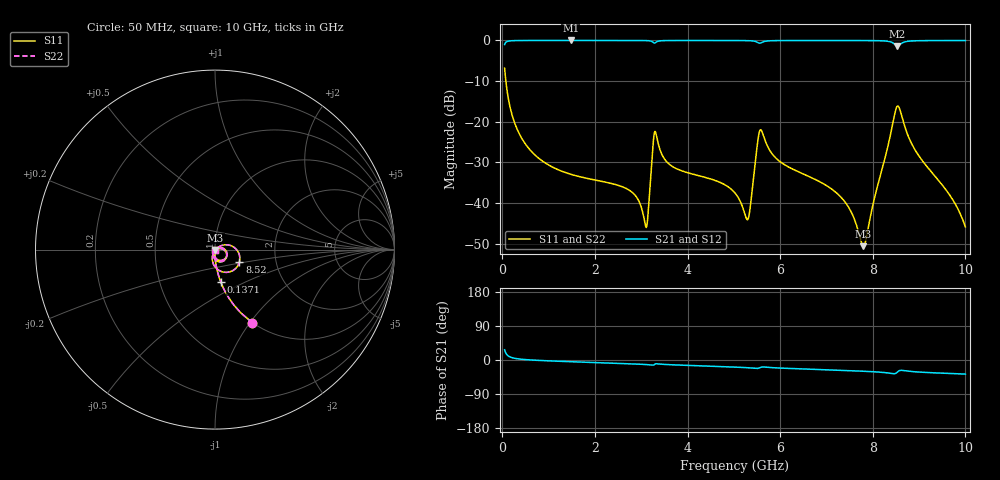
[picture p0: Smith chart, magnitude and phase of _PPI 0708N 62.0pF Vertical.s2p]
! S-Parameter data specifications (vertical orientation):
! Substrate: 40-mil Rogers 3003C, Substrate thickness, H=1.016mm, Dielectric constant, Er=3, Conductor thickness, T_mtl=0.043mm, Loss Tangent, Tand=0.003
! PCB Mounting Pad Footprint: Pad width, PadW=2.54mm , Pad length, PadL=0.51mm , Pad gap, PadG (edge-to-edge)=0.71mm , Reference planes=1.73mm apart
! Created Tue Jan 16 08:53:59 2018
# GHz S MA R 50
! 2 Port Network Data from SP1.SP block
! freq  magS11  angS11  magS21  angS21  magS12  angS12  magS22  angS22
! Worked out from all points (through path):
!   801 points, 50 MHz to 10 GHz, reference 50 ohm
!   highest |S21| = -0.01 dB at 1.48 GHz (marker M1); lowest = -1.5 dB at 8.532 GHz (marker M2)
!   group delay of S21, straight-line fit = 11.1 ps
!   lowest |S11| = -50.6 dB at 7.799 GHz (marker M3), VSWR 1.01, Z = 50.2 - j0.181 ohm
!   |S11| at or under -10 dB: 76.96 MHz to end of sweep
!   |S22| runs from -50.6 to -6.8 dB; largest |S21 - S12| = 0
!   S11 on the Smith chart (normalised r, x): 50 MHz: 1.00, -1.02; 137.1 MHz: 1.00, -0.37; 8.52 GHz: 1.30, -0.19; 10 GHz: 1.00, -0.01
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0.05  0.4558 -63.1  0.8899 26.9  0.8899 26.9  0.4558 -63.1
0.1370625  0.1841 -79.9  0.9827 10.1  0.9827 10.1  0.1841 -79.9
0.572375  0.04687 -89.2  0.9986 0.4  0.9986 0.4  0.04687 -89.2
1.480312  0.02255 -93.4  0.9992 -4.5  0.9992 -4.5  0.02255 -93.4
1.716625  0.02077 -94.2  0.9992 -5.5  0.9992 -5.5  0.02077 -94.2
2.761375  0.01412 -96.1  0.9988 -10.0  0.9988 -10.0  0.01412 -96.1
3.097187  0.00511 -49.2  0.9958 -11.9  0.9958 -11.9  0.00511 -49.2
3.271313  0.06504 -9.0  0.935 -13.0  0.935 -13.0  0.06504 -9.0
3.370812  0.0528 -81.0  0.9811 -10.3  0.9811 -10.3  0.0528 -81.0
3.669313  0.02822 -98.6  0.9975 -12.7  0.9975 -12.7  0.02822 -98.6
5.025  0.01327 -100.0  0.9977 -18.7  0.9977 -18.7  0.01327 -100.0
5.311063  0.006412 -33.8  0.9935 -20.4  0.9935 -20.4  0.006412 -33.8
5.584688  0.07944 -52.0  0.9322 -19.1  0.9322 -19.1  0.07944 -52.0
5.932938  0.03455 -104.0  0.995 -20.9  0.995 -20.9  0.03455 -104.0
6.691625  0.02031 -109.8  0.9978 -24.5  0.9978 -24.5  0.02031 -109.8
7.388125  0.01051 -107.2  0.9977 -27.6  0.9977 -27.6  0.01051 -107.2
7.798563  0.002942 -37.8  0.9968 -29.7  0.9968 -29.7  0.002942 -37.8
8.345812  0.05558 27.6  0.9724 -34.5  0.9724 -34.5  0.05558 27.6
8.519937  0.153 -27.2  0.8473 -33.2  0.8473 -33.2  0.153 -27.2
8.532375  0.156 -34.9  0.8438 -31.8  0.8438 -31.8  0.156 -34.9
8.9055  0.04573 -109.0  0.9891 -31.1  0.9891 -31.1  0.04573 -109.0
10  0.005078 -101.5  0.9974 -37.2  0.9974 -37.2  0.005078 -101.5
